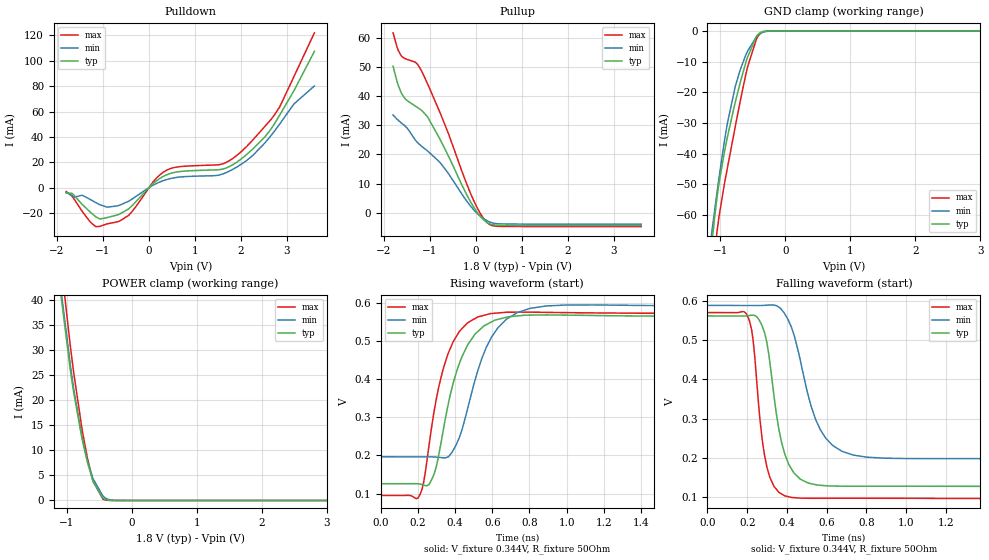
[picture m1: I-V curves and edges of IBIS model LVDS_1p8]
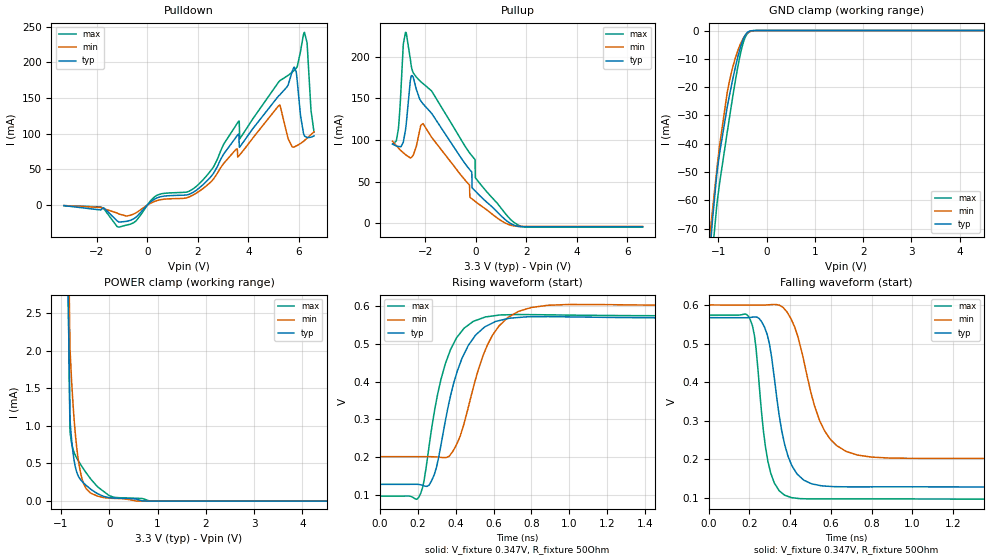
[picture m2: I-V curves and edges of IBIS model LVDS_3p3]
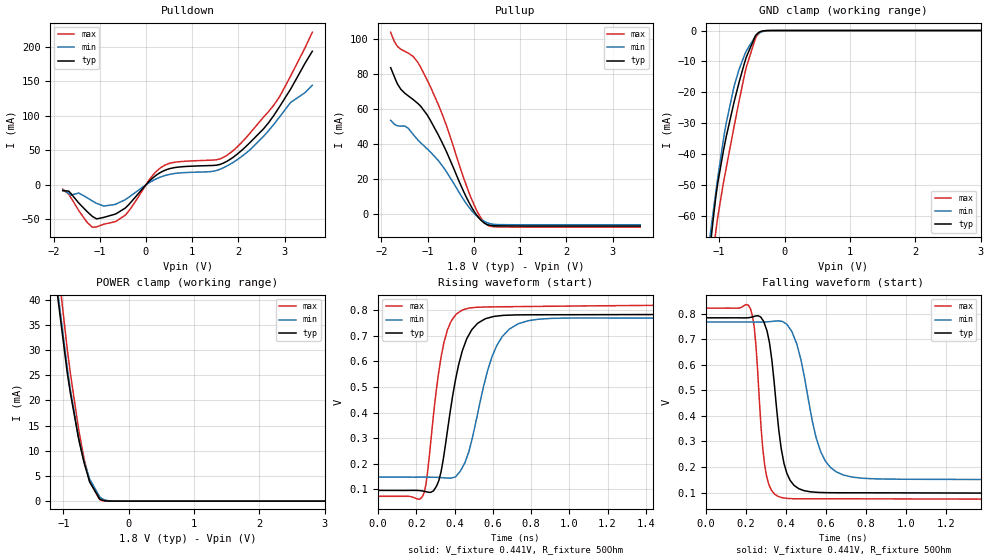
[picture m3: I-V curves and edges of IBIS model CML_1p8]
| Texas Instruments Incorporated
| Ultra-Low Jitter Clock Synchronizer and Jitter Cleaner with Two
| Frequency Domains, Eight Differential Outputs, Two Differential Inputs
[IBIS Ver]   4.1
[File name]   lmk05318.ibs
[Date]   05/15/2018
[File Rev]   1.0
[Source]
| Texas Instruments Incorporated.
| Analog-eLab Design Center, HPA
| 12500 TI Blvd
| Dallas, TX -75243
[Notes]   Revision History:
| Rev 1.0: 05/15/2018
| - Initial version of the model
| - Model generated from simulations in SPECTRE
| - C_comp although listed in numerical order of value are
|   obtained from varying PVT conditions. For PVT conditions for
|   each specific value refer the buffer description under
|   respective [Model]. IBIS model user is responsible for using
|   appropriate C_comp to simulate for Signal Integrity.
| - Warnings regarding combined Non-monotonicity of various models
|   have been reviewed and considered minor and can be ignored.
| - Model names with a trailing _1p8 contain the model for
|   1.8V operation. Model names with a trailing _2p5 contain the model
|   for 2.5V operation. Model names with a trailing _3p3 contain the model
|   for 3.3V operation.
| - INX Model: Differential Input buffer normally driven differentially,
|   but can be driven with single ended signal. Comment out particular pin numbers
|   in [Diff pin] section to configure the pins as single-ended input.
| - INX Model: Model generated with internal termination resistors disabled. Use
|   100 Ohm differential termination or 50 Ohm to ground termination in user's
|   simulation set up.
| - xo Model: Differential Input buffer normally driven differentially,
|   but can be driven with single ended signal. Comment out particular pin numbers
|   in [Diff pin] section to configure the pins as single-ended input.
| - xo Model: Model generated with internal termination resistors disabled. Use
|   100 Ohm differential termination or 50 Ohm to ground termination in user's
|   simulation set up.
[Disclaimer]
| This model is designed as an aid for customers of Texas Instruments.
| TI and its licensors and suppliers make no warranties, either expressed
| or implied, with respect to this  model, including the warranties of
| merchantability or fitness for a particular purpose. The model is
| provided solely on an "as is" basis. The entire risk as to its quality
| and performance is with the customer.
| This model is subject to change without notice. Texas Instruments
| Incorporated is not responsible for updating this model.
[Copyright]
(C) Copyright 2018 Texas Instruments Incorporated.All rights reserved.
|  Component LMK05318RGZ 48-pin QFN - RGZ package
|  Part # LMK05318RGZ
[Component]   LMK05318RGZ
[Manufacturer]  TI
[Package]   |48 QFN - RGZ package
|   typ   min   max
R_pkg   0.05   0.04   0.06
L_pkg   1.0nH   0.8nH   1.2nH
C_pkg   0.2pF   0.16pF   0.24pF
[Pin]  signal_name   model_name   R_pin   L_pin   C_pin
1   STATUS0   GPIO   NA   NA   NA
2   STATUS1   GPIO   NA   NA   NA
3   CAP_DIG   nc   NA   NA   NA
4   VDD_DIG   power   NA   NA   NA
5   VDD_IN   power   NA   NA   NA
6   PRIREF_P   INX   NA   NA   NA
7   PRIREF_N   INX   NA   NA   NA
8   REFSEL   nc   NA   NA   NA
9   HW_SW_CTRL   nc   NA   NA   NA
10   SECREF_P   INX   NA   NA   NA
11   SECREF_N   INX   NA   NA   NA
12   GPIO0   GPIO   NA   NA   NA
13   PDN   nc   NA   NA   NA
14   OUT0_P   diffout   NA   NA   NA
15   OUT0_N   diffout   NA   NA   NA
16   OUT1_N   diffout   NA   NA   NA
17   OUT1_P   diffout   NA   NA   NA
18   VDDO_01   power   NA   NA   NA
19   VDDO_23   power   NA   NA   NA
20   OUT2_P   diffout   NA   NA   NA
21   OUT2_N   diffout   NA   NA   NA
22   OUT3_N   diffout   NA   NA   NA
23   OUT3_P   diffout   NA   NA   NA
24   GPIO1   GPIO   NA   NA   NA
25   SDA   I2C   NA   NA   NA
26   SCL   I2C   NA   NA   NA
27   VDD_PLL1   power   NA   NA   NA
28   CAP_PLL1   nc   NA   NA   NA
29   LF1   nc   NA   NA   NA
30   GPIO2   GPIO   NA   NA   NA
31   XO_P   xo   NA   NA   NA
32   XO_N   xo   NA   NA   NA
33   VDD_XO   power   NA   NA   NA
34   LF2   nc   NA   NA   NA
35   CAP_PLL2   nc   NA   NA   NA
36   VDD_PLL2   power   NA   NA   NA
37   VDDO_4   power   NA   NA   NA
38   OUT4_N   diffout1   NA   NA   NA
39   OUT4_P   diffout1   NA   NA   NA
40   VDDO_5   power   NA   NA   NA
41   OUT5_N   diffout1   NA   NA   NA
42   OUT5_P   diffout1   NA   NA   NA
43   VDDO_6   power   NA   NA   NA
44   OUT6_N   diffout1   NA   NA   NA
45   OUT6_P   diffout1   NA   NA   NA
46   VDDO_7   power   NA   NA   NA
47   OUT7_N   diffout1   NA   NA   NA
48   OUT7_P   diffout1   NA   NA   NA
[Diff pin]  inv_pin  vdiff  tdelay_typ  tdelay_min  tdelay_max
6   7   0.2   0.0s   0.0s   0.0s
10   11   0.2   0.0s   0.0s   0.0s
14   15   0.0   0.0s   0.0s   0.0s
17   16   0.0   0.0s   0.0s   0.0s
20   21   0.0   0.0s   0.0s   0.0s
23   22   0.0   0.0s   0.0s   0.0s
31   32   0.2   0.0s   0.0s   0.0s
39   38   0.0   0.0s   0.0s   0.0s
42   41   0.0   0.0s   0.0s   0.0s
45   44   0.0   0.0s   0.0s   0.0s
48   47   0.0   0.0s   0.0s   0.0s
|   Model Selectors
[Model Selector] diffout
LVDS_1p8   1.8V   LVDS
LVDS_3p3   3.3V   LVDS
CML_1p8   1.8V   CML
CML_3p3   3.3V   CML
LVPECL_1p8   1.8V   LVPECL
LVPECL_3p3   3.3V   LVPECL
HCSL_1p8   1.8V   HCSL
HCSL_3p3   3.3V   HCSL
[Model Selector] diffout1
LVDS_1p8   1.8V   LVDS
LVDS_3p3   3.3V   LVDS
CML_1p8   1.8V   CML
CML_3p3   3.3V   CML
LVPECL_1p8   1.8V   LVPECL
LVPECL_3p3   3.3V   LVPECL
HCSL_1p8   1.8V   HCSL
HCSL_3p3   3.3V   HCSL
LVCMOS_FAST_1p8   1.8V   LVCMOS
[Model Selector] GPIO
GPIO_IO   3.3V   digital I/O
GPIO_OD   3.3V   digital Open_drain
| Models and submodels in the file (14): LVDS_1p8 (3-state), LVDS_3p3 (3-state), CML_1p8 (3-state), CML_3p3 (3-state), LVPECL_1p8 (3-state), LVPECL_3p3 (3-state), HCSL_1p8 (Open_source), HCSL_3p3 (Open_source), LVCMOS_FAST_1p8 (3-state), GPIO_IO (I/O), GPIO_OD (I/O_open_drain), I2C (I/O_open_drain), xo (Input), INX (Input)
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|   LVDS_1p8 Model
[Model]   LVDS_1p8
Model_type   3-state
Polarity   Non-Inverting
Vmeas = 0.344
Vref = 0.344
Cref = 2pF
Rref = 50
|   typ   min   max
C_comp   1.5263E-12   1.43105E-12   1.63546E-12
| Where nom  PVT is Nominal Process, 1.8V, 27C
|   Fast PVT is Strong Process,  1.9V, -40C
|   Slow PVT is Weak Process,   1.7V, 125C
[Voltage Range]   1.8   1.7   1.9
|Junction Temperature
[Temperature Range]   27   125   -40
[Pullup Reference]   1.8   1.7   1.9
[Pulldown Reference]   0   -0   0
[Power Clamp Reference]   1.8   1.7   1.9
[GND Clamp Reference]   0   0   0
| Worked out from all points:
|   slope of the pulldown table from 0 to 0.27 V, typ, clamps not added: 33.7 ohm
|   slope of the pullup table from 0 to 0.27 V, typ, clamps not added: 60.8 ohm
|   GND clamp passes 1 mA (typ) near -0.42 V on its own axis
|   POWER clamp passes 1 mA (typ) near -0.47 V on its own axis
|   falling waveform, V_fixture 0.344V, R_fixture 50Ohm: 20-80 % time 81.9ps typ, 127ps min, 58.9ps max; typ from 0.562 V to 0.126 V
|   rising waveform, V_fixture 0.344V, R_fixture 50Ohm: 20-80 % time 137ps typ, 156ps min, 121ps max; typ from 0.126 V to 0.562 V
[Pulldown]
|   Voltage   I(typ)   I(min)   I(max)
-1.8V     -4.239mA   -3.713mA   -3.012mA
-1.665V   -4.76mA    -6.39mA    -7.11mA
-1.271V   -19.43mA   -9.399mA   -27.25mA
-1.071V   -24.6mA    -13.37mA   -30.52mA
-444.6mV  -16.77mA   -10.72mA   -21.92mA
106.2mV   3.721mA    2.27mA     5.207mA
387mV     10.18mA    6.441mA    13.83mA
1.753V    16.7mA     13.13mA    21.36mA
2.25V     30.2mA     25.16mA    37.2mA
2.731V    50.33mA    44.52mA    57.33mA
3.146V    75.89mA    65.6mA     86.87mA
3.6V      107.4mA    80.15mA    122mA
[GND Clamp]
|   Voltage   I(typ)   I(min)   I(max)
-1.8V     -227.5mA   -244.3mA   -293.8mA
-1.125V   -67.81mA   -64.27mA   -79.09mA
-1.114V   -65.59mA   -62.48mA   -76.82mA
-1.093V   -61.33mA   -58.94mA   -72.53mA
-1.049V   -53.68mA   -52.02mA   -64.8mA
-909mV    -36.18mA   -32mA      -46.42mA
-768.6mV  -22.88mA   -17.82mA   -30.77mA
-585mV    -8.613mA   -6.634mA   -11.87mA
-444.6mV  -1.694mA   -1.777mA   -2.489mA
-385.2mV  -510.7uA   -772.5uA   -830.7uA
-217.8mV  -3.668uA   -26.55uA   -3.583uA
3.6V      0A         0A         0A
[Pullup]
|   Voltage   I(typ)   I(min)   I(max)
-1.8V     50.26mA    33.56mA    61.75mA
-1.692V   43.98mA    31.79mA    55.91mA
-1.579V   39.99mA    30.29mA    53.25mA
-1.309V   36.53mA    24.8mA     51.58mA
-1.163V   34.9mA     22.62mA    48.14mA
-1.044V   32.77mA    21.15mA    44.08mA
-757.8mV  24.57mA    16.83mA    33.57mA
-104.4mV  3.511mA    2.097mA    6.286mA
84.6mV    -973.8uA   -993.9uA   134.7uA
262.8mV   -3.54mA    -2.879mA   -3.598mA
516.6mV   -4.275mA   -3.817mA   -4.674mA
3.6V      -4.356mA   -3.909mA   -4.758mA
[POWER Clamp]
|   Voltage   I(typ)   I(min)   I(max)
-1.8V     167.1mA    290.8mA    175.6mA
-1.103V   42.32mA    43.41mA    48.96mA
-941.4mV  25.56mA    26.6mA     30.29mA
-892.8mV  21.47mA    22.2mA     25.41mA
-774mV    12.9mA     13.11mA    14.91mA
-752.4mV  11.54mA    11.74mA    13.24mA
-682.2mV  7.588mA    7.904mA    8.398mA
-595.8mV  3.783mA    4.344mA    3.83mA
-444.6mV  459.2uA    875.5uA    303.4uA
-352.8mV  57.32uA    198.5uA    23.38uA
-217.8mV  991nA      11.87uA    112.9nA
3.6V      0A         0A         0A
[Ramp]
R_load = 50
|   typ   min   max
dV/dt_r   0.261621/1.36673e-10   0.235532/1.55726e-10   0.285144/1.20651e-10
dV/dt_f   0.261698/8.18668e-11   0.235475/1.27479e-10   0.285181/5.89491e-11
[Falling Waveform]
V_fixture = 0.344V
V_fixture_min = 0.392V
V_fixture_max = 0.333V
R_fixture = 50Ohm
C_fixture = 0F
|   Time   V(typ)   V(min)   V(max)
0s        562.3mV    589.2mV    570.7mV
201.4ps   562.6mV    588.9mV    562.3mV
230.2ps   564.1mV    588.8mV    498.3mV
264.5ps   547.8mV    588.8mV    296.5mV
299ps     494.3mV    589.7mV    176.7mV
359.4ps   272.8mV    584.7mV    111.9mV
390.1ps   207.9mV    566.6mV    102.6mV
544.8ps   131.2mV    297.2mV    96.48mV
676.5ps   127.3mV    216.5mV    96.61mV
2.5ns     126.1mV    196.7mV    95.44mV
[Rising Waveform]
V_fixture = 0.344V
V_fixture_min = 0.392V
V_fixture_max = 0.333V
R_fixture = 50Ohm
C_fixture = 0F
|   Time   V(typ)   V(min)   V(max)
0s        126.2mV    196.5mV    95.4mV
201.4ps   126mV      196.4mV    89.02mV
260.2ps   124.1mV    196.4mV    226.6mV
298.4ps   169.5mV    195.8mV    345.4mV
360.5ps   327.7mV    196mV      463.8mV
434.6ps   455.6mV    263.7mV    530.4mV
522.8ps   524.3mV    422.8mV    562.5mV
630.1ps   555.8mV    533.8mV    572.7mV
802.6ps   567mV      584.7mV    574.8mV
2.5ns     562.2mV    589.1mV    570.6mV
|   LVDS_3p3 Model
[Model]   LVDS_3p3
Model_type   3-state
Polarity   Non-Inverting
Vmeas = 0.347
Vref = 0.347
Cref = 2pF
Rref = 50
|   typ   min   max
C_comp   1.41794E-12   1.36037E-12   1.45091E-12
| Where nom  PVT is Nominal Process, 3.3V, 27C
|   Fast PVT is Strong Process,  3.45V, -40C
|   Slow PVT is Weak Process,   3.15V, 125C
[Voltage Range]   3.3   3.15   3.45
|Junction Temperature
[Temperature Range]   27   125   -40
[Pullup Reference]   3.3   3.15   3.45
[Pulldown Reference]   0   0   0
[Power Clamp Reference]   3.3   3.15   3.45
[GND Clamp Reference]   0   0   0
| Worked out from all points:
|   slope of the pulldown table from 0 to 0.495 V, typ, clamps not added: 43.3 ohm
|   slope of the pullup table from 0 to 0.495 V, typ, clamps not added: 34.5 ohm
|   GND clamp passes 1 mA (typ) near -0.41 V on its own axis
|   POWER clamp passes 1 mA (typ) near -0.80 V on its own axis
|   falling waveform, V_fixture 0.347V, R_fixture 50Ohm: 20-80 % time 81ps typ, 126ps min, 58ps max; typ from 0.567 V to 0.127 V
|   rising waveform, V_fixture 0.347V, R_fixture 50Ohm: 20-80 % time 134ps typ, 152ps min, 119ps max; typ from 0.127 V to 0.567 V
[Pulldown]
|   Voltage   I(typ)   I(min)   I(max)
-3.3V     -682.7uA   -556.3uA   -680.5uA
-1.845V   -6.734mA   -3.237mA   -2.416mA
-1.122V   -23.79mA   -12.43mA   -30.82mA
382.8mV   10.12mA    6.397mA    13.75mA
1.798V    17.55mA    13.9mA     22.39mA
3.61V     99.56mA    68.31mA    117.2mA
5.234V    154.2mA    140.1mA    173.8mA
5.818V    193.5mA    81.61mA    189mA
6.224V    96.88mA    90.66mA    242.2mA
6.323V    94.68mA    93.82mA    228mA
6.481V    95.17mA    98.89mA    132.9mA
6.6V      96.99mA    102.7mA    102.3mA
[GND Clamp]
|   Voltage   I(typ)   I(min)   I(max)
-3.3V     -1.225A    -1.029A    -1.515A
-1.181V   -80.15mA   -73.74mA   -92.54mA
-1.132V   -69.26mA   -65.41mA   -80.58mA
-1.122V   -67.19mA   -63.77mA   -78.45mA
-1.033V   -51.11mA   -49.44mA   -62.14mA
-973.5mV  -43.33mA   -40.6mA    -53.92mA
-815.1mV  -26.99mA   -21.86mA   -35.94mA
-765.6mV  -22.62mA   -17.58mA   -30.43mA
-528mV    -5.185mA   -4.26mA    -7.227mA
-438.9mV  -1.534mA   -1.654mA   -2.27mA
-349.8mV  -210.4uA   -427.7uA   -364.9uA
6.6V      0A         0A         0A
[Pullup]
|   Voltage   I(typ)   I(min)   I(max)
-3.3V     95.18mA    98.51mA    95.14mA
-3.072V   92.32mA    90.66mA    112.5mA
-2.874V   97.38mA    84.73mA    215.2mA
-2.785V   112.5mA    82.48mA    229.6mA
-2.528V   177.5mA    79.85mA    184.7mA
-2.092V   143.5mA    119.8mA    167.9mA
-250.8mV  64.63mA    45.78mA    84.63mA
-231mV    63.91mA    31.05mA    83.82mA
-33mV     38.92mA    26.3mA     76.47mA
-23.1mV   38.61mA    26.07mA    54.68mA
1.492V    -2.189mA   -3.282mA   1.328mA
6.6V      -4.397mA   -3.974mA   -4.785mA
[POWER Clamp]
|   Voltage   I(typ)   I(min)   I(max)
-3.3V     2.746A     3.266A     2.249A
-1.488V   31.11mA    34.76mA    35.04mA
-815.1mV  1.082mA    2.027mA    921.9uA
-775.5mV  776.3uA    1.532mA    752.1uA
-726mV    528.1uA    1.059mA    641.3uA
-627mV    314.2uA    482.9uA    520.1uA
-557.7mV  256.3uA    280uA      449.6uA
-478.5mV  207.7uA    164.7uA    374.7uA
-260.7mV  105.7uA    70.86uA    202.7uA
75.9mV    41.45uA    37.03uA    56.03uA
897.6mV   0A         127.3nA    190.5nA
6.6V      0A         0A         0A
[Ramp]
R_load = 50
|   typ   min   max
dV/dt_r   0.264018/1.34056e-10   0.239697/1.51904e-10   0.286831/1.18584e-10
dV/dt_f   0.264093/8.09643e-11   0.239603/1.25829e-10   0.286868/5.79709e-11
[Falling Waveform]
V_fixture = 0.347V
V_fixture_min = 0.4V
V_fixture_max = 0.335V
R_fixture = 50Ohm
C_fixture = 0F
|   Time   V(typ)   V(min)   V(max)
0s        567.4mV    600.4mV    574.2mV
204.2ps   568mV      600.1mV    562.3mV
232.6ps   569.1mV    600.1mV    488.2mV
269ps     548.2mV    600.1mV    273.1mV
291ps     515.7mV    600.7mV    194.3mV
373.1ps   238.3mV    589.3mV    106.8mV
433.8ps   162mV      524.9mV    98.67mV
544.4ps   132.1mV    300.9mV    97.08mV
675.2ps   128.5mV    220.3mV    97.21mV
2.5ns     127.3mV    201.1mV    96.05mV
[Rising Waveform]
V_fixture = 0.347V
V_fixture_min = 0.4V
V_fixture_max = 0.335V
R_fixture = 50Ohm
C_fixture = 0F
|   Time   V(typ)   V(min)   V(max)
0s        127.3mV    200.8mV    96.01mV
204.2ps   127mV      200.7mV    92.42mV
260ps     125.4mV    200.7mV    230.7mV
298.2ps   172.1mV    200.1mV    349.9mV
345.7ps   296.7mV    198.3mV    448.2mV
422.6ps   447.4mV    253.8mV    528.1mV
492.9ps   514.9mV    383.7mV    560.1mV
628.7ps   562mV      547.7mV    576.7mV
800.4ps   572.3mV    597.1mV    578mV
2.5ns     567.3mV    600.3mV    574.1mV
|   CML_1p8 Model
[Model]   CML_1p8
Model_type   3-state
Polarity   Non-Inverting
Vmeas = 0.441
Vref = 0.441
Cref = 2pF
Rref = 50
|   typ   min   max
C_comp   1.5263E-12   1.43105E-12   1.63546E-12
| Where nom  PVT is Nominal Process, 1.8V, 27C
|   Fast PVT is Strong Process,  1.9V, -40C
|   Slow PVT is Weak Process,   1.7V, 125C
[Voltage Range]   1.8   1.7   1.9
|Junction Temperature
[Temperature Range]   27   125   -40
[Pullup Reference]   1.8   1.7   1.9
[Pulldown Reference]   0   0   0
[Power Clamp Reference]   1.8   1.7   1.9
[GND Clamp Reference]   0   0   0
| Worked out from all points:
|   slope of the pulldown table from 0 to 0.27 V, typ, clamps not added: 16.8 ohm
|   slope of the pullup table from 0 to 0.27 V, typ, clamps not added: 35.7 ohm
|   GND clamp passes 1 mA (typ) near -0.42 V on its own axis
|   POWER clamp passes 1 mA (typ) near -0.47 V on its own axis
|   falling waveform, V_fixture 0.441V, R_fixture 50Ohm: 20-80 % time 60.8ps typ, 102ps min, 40.9ps max; typ from 0.784 V to 0.096 V
|   rising waveform, V_fixture 0.441V, R_fixture 50Ohm: 20-80 % time 99ps typ, 127ps min, 77.2ps max; typ from 0.096 V to 0.784 V
[Pulldown]
|   Voltage   I(typ)   I(min)   I(max)
-1.8V     -8.523mA   -7.443mA   -6.058mA
-1.665V   -9.59mA    -12.82mA   -14.31mA
-1.271V   -38.91mA   -18.85mA   -54.56mA
-1.071V   -49.24mA   -26.78mA   -61.08mA
-444.6mV  -33.56mA   -21.46mA   -43.87mA
106.2mV   7.449mA    4.544mA    10.42mA
387mV     20.38mA    12.9mA     27.68mA
1.748V    33.93mA    27.12mA    42.58mA
2.261V    61.9mA     51.39mA    75.63mA
2.763V    100.2mA    87.31mA    115.2mA
3.13V     138.7mA    119.3mA    157.7mA
3.6V      193.6mA    144.3mA    221mA
[GND Clamp]
|   Voltage   I(typ)   I(min)   I(max)
-1.8V     -227.5mA   -244.3mA   -293.8mA
-1.125V   -67.81mA   -64.27mA   -79.09mA
-1.114V   -65.59mA   -62.48mA   -76.82mA
-1.093V   -61.33mA   -58.94mA   -72.53mA
-1.049V   -53.68mA   -52.02mA   -64.8mA
-909mV    -36.18mA   -32mA      -46.42mA
-768.6mV  -22.88mA   -17.82mA   -30.77mA
-585mV    -8.613mA   -6.634mA   -11.87mA
-444.6mV  -1.694mA   -1.777mA   -2.489mA
-385.2mV  -510.7uA   -772.5uA   -830.7uA
-217.8mV  -3.668uA   -26.55uA   -3.583uA
3.6V      0A         0A         0A
[Pullup]
|   Voltage   I(typ)   I(min)   I(max)
-1.8V     83.56mA    53.51mA    103.7mA
-1.676V   75.54mA    50.61mA    96.51mA
-1.584V   71.38mA    50.19mA    94.17mA
-1.422V   67.5mA     48.97mA    91.92mA
-1.314V   65.37mA    45.43mA    89.99mA
-1.012V   56.64mA    37.22mA    76.57mA
-617.4mV  36.99mA    25.08mA    52.29mA
-61.2mV   4.438mA    2.328mA    9.261mA
133.2mV   -3.017mA   -2.667mA   -1.413mA
268.2mV   -5.807mA   -4.779mA   -5.856mA
538.2mV   -6.787mA   -6.078mA   -7.418mA
3.6V      -6.9mA     -6.194mA   -7.536mA
[POWER Clamp]
|   Voltage   I(typ)   I(min)   I(max)
-1.8V     167.1mA    290.8mA    175.6mA
-1.103V   42.32mA    43.41mA    48.96mA
-941.4mV  25.56mA    26.6mA     30.29mA
-892.8mV  21.47mA    22.2mA     25.41mA
-774mV    12.9mA     13.11mA    14.91mA
-752.4mV  11.54mA    11.74mA    13.24mA
-682.2mV  7.588mA    7.904mA    8.398mA
-595.8mV  3.783mA    4.344mA    3.83mA
-444.6mV  459.2uA    875.5uA    303.4uA
-352.8mV  57.32uA    198.5uA    23.38uA
-217.8mV  991nA      11.87uA    112.9nA
3.6V      0A         0A         0A
[Ramp]
R_load = 50
|   typ   min   max
dV/dt_r   0.412396/9.90447e-11   0.371599/1.27393e-10   0.449009/7.71613e-11
dV/dt_f   0.412547/6.07842e-11   0.371457/1.01535e-10   0.449065/4.09336e-11
[Falling Waveform]
V_fixture = 0.441V
V_fixture_min = 0.458V
V_fixture_max = 0.449V
R_fixture = 50Ohm
C_fixture = 0F
|   Time   V(typ)   V(min)   V(max)
0s        783.8mV    767.6mV    821.8mV
222.5ps   785.7mV    767.5mV    817.7mV
249.8ps   791.1mV    767.3mV    671mV
292.8ps   759.2mV    767.7mV    208.1mV
328.9ps   618.8mV    769.8mV    106.3mV
362.4ps   353.9mV    771.7mV    84.06mV
439.5ps   128.3mV    709.4mV    75.65mV
572.9ps   100.1mV    260.2mV    75.46mV
686.7ps   99.01mV    168.4mV    75.4mV
2.5ns     96.26mV    148.6mV    73.31mV
[Rising Waveform]
V_fixture = 0.441V
V_fixture_min = 0.458V
V_fixture_max = 0.449V
R_fixture = 50Ohm
C_fixture = 0F
|   Time   V(typ)   V(min)   V(max)
0s        96.39mV    148.3mV    73.27mV
232.5ps   94.1mV     148.1mV    74.1mV
257.6ps   90.05mV    148.1mV    162.9mV
305.3ps   113.1mV    147.5mV    494.4mV
344.4ps   237.2mV    145.5mV    674.9mV
439.5ps   639.5mV    185mV      800mV
489.5ps   723.4mV    291.8mV    808.8mV
595.1ps   773.2mV    617.3mV    812.3mV
730.2ps   781.1mV    745.7mV    813.4mV
2.5ns     783.7mV    767.6mV    821.6mV
